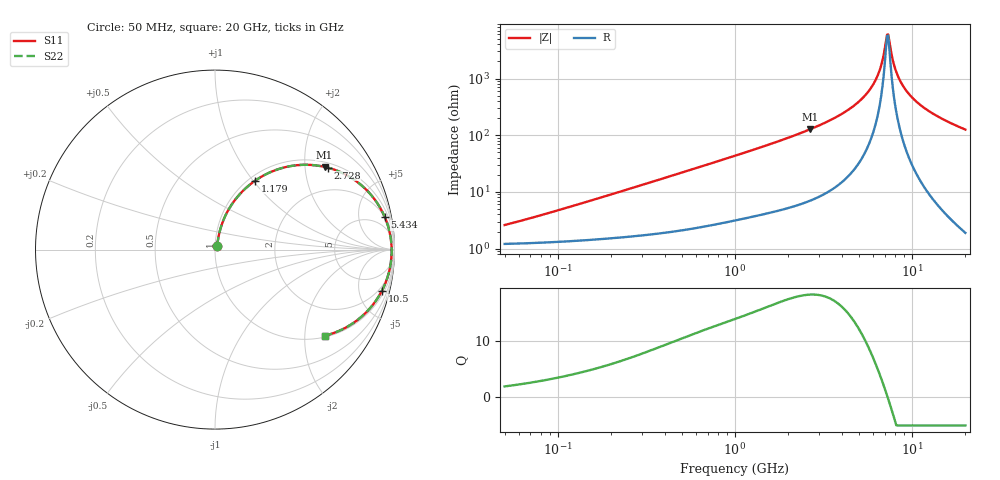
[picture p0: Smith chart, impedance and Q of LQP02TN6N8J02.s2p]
!Murata Part Number: LQP02TN6N8J02
!These Parameters are Measured in Series Mode Connection
!  o--[Z]--o
!Port1  Port2
!  o-------o
!Freq. Start=50[MHz] Stop=20[GHz], 401[Steps]
# Hz S RI R 50
!Freq.(Hz) S11(Real) S11(Imag) S21(Real) S21(Imag) S12(Real) S12(Imag) S22(Real) S22(Imag)
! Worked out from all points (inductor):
!   401 points, 50 MHz to 20 GHz, reference 50 ohm
!   read as one part in series: L = 7.22 nH near 84.46 MHz
!   highest Q = 18.2 at 2.647 GHz (marker M1), where L = 7.6 nH
!   self-resonance near 7.222 GHz
!   S11 on the Smith chart (normalised r, x): 50 MHz: 1.02, +0.05; 1.179 GHz: 1.07, +1.02; 2.728 GHz: 1.14, +2.63; 5.434 GHz: 2, +10; 10.5 GHz: 1.43, -7.97; 20 GHz: 1.04, -2.51
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5e7  0.0125 0.0225  0.9875 -0.0225  0.9875 -0.0225  0.0125 0.0225
1.364002e8  0.0173 0.0595  0.9827 -0.0595  0.9827 -0.0595  0.0173 0.0595
3.721004e8  0.0426 0.1533  0.9574 -0.1533  0.9574 -0.1533  0.0426 0.1533
1e9  0.1757 0.3461  0.8243 -0.3461  0.8243 -0.3461  0.1757 0.3461
1.179116e9  0.2236 0.384  0.7764 -0.384  0.7764 -0.384  0.2236 0.384
1.875929e9  0.4183 0.4649  0.5817 -0.4649  0.5817 -0.4649  0.4183 0.4649
2.647493e9  0.6101 0.461  0.3899 -0.461  0.3899 -0.461  0.6101 0.461
2.728004e9  0.6275 0.4568  0.3725 -0.4568  0.3725 -0.4568  0.6275 0.4568
4.087748e9  0.8435 0.333  0.1565 -0.333  0.1565 -0.333  0.8435 0.333
5.433528e9  0.9453 0.183  0.0547 -0.183  0.0547 -0.183  0.9453 0.183
5.944466e9  0.9649 0.1286  0.0351 -0.1286  0.0351 -0.1286  0.9649 0.1286
6.406762e9  0.9761 0.0817  0.0239 -0.0817  0.0239 -0.0817  0.9761 0.0817
6.701223e9  0.9805 0.0531  0.0195 -0.0531  0.0195 -0.0531  0.9805 0.0531
7.114996e9  0.9838 0.0146  0.0162 -0.0146  0.0162 -0.0146  0.9838 0.0146
7.222371e9  0.9841 0.00493  0.0159 -0.00493  0.0159 -0.00493  0.9841 0.00493
7.442007e9  0.9842 -0.0144  0.0158 0.0144  0.0158 0.0144  0.9842 -0.0144
7.901521e9  0.982 -0.0531  0.018 0.0531  0.018 0.0531  0.982 -0.0531
8.389408e9  0.9767 -0.0915  0.0233 0.0915  0.0233 0.0915  0.9767 -0.0915
9.178299e9  0.9631 -0.1483  0.0369 0.1483  0.0369 0.1483  0.9631 -0.1483
1.050288e10  0.9299 -0.2296  0.0701 0.2296  0.0701 0.2296  0.9299 -0.2296
1.396067e10  0.8149 -0.3751  0.1851 0.3751  0.1851 0.3751  0.8149 -0.3751
2e10  0.6106 -0.4801  0.3894 0.4801  0.3894 0.4801  0.6106 -0.4801
